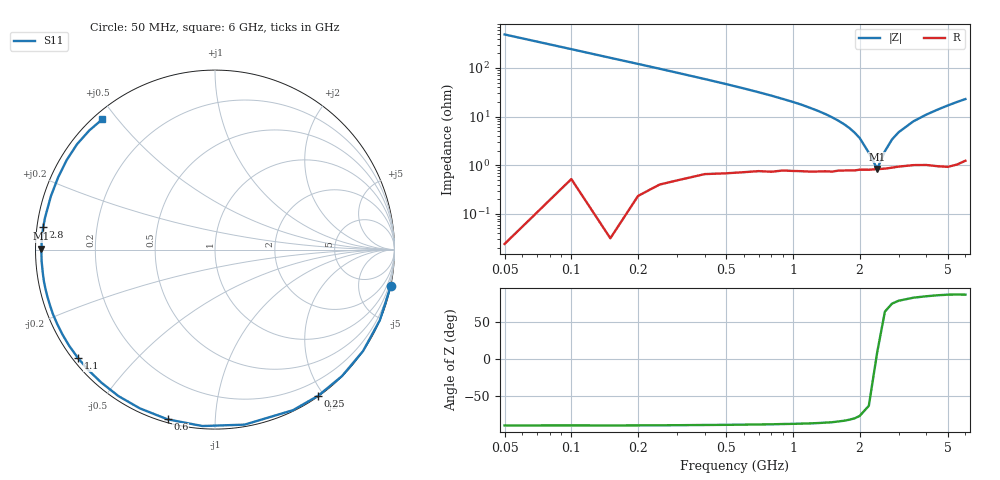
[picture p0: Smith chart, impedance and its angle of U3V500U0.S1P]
! SIEMENS Discrete & RF Semiconductors
! BBY53-02W
! Si Tuning Diode in SCD-80
! VR = 0.5 V
! S-Parameters:  September  1997
# GHz  S  MA  R  50
!  f  S11
! GHz  MAG  ANG
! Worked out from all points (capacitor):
!   34 points, 50 MHz to 6 GHz, reference 50 ohm
!   read as one part to ground: C = 6.52 pF near 50 MHz
!   lowest |Z| = 840 mohm at 2.4 GHz (marker M1)
!   series resonance near 2.385 GHz, so ESL is about 680 pH
!   S11 on the Smith chart (normalised r, x): 50 MHz: 0.00, -9.76; 250 MHz: 0.01, -1.93; 600 MHz: 0.01, -0.76; 1.1 GHz: 0.02, -0.35; 2.8 GHz: 0.02, +0.07; 6 GHz: 0.02, +0.46
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0.05  1 -11.7
0.1  0.9992 -23.2
0.15  0.9999 -34.4
0.2  0.9986 -44.9
0.25  0.9966 -54.8
0.3  0.9945 -64.1
0.4  0.9891 -80.4
0.5  0.9855 -94.1
0.6  0.9819 -105.6
0.7  0.9787 -115.3
0.8  0.9775 -123.4
0.9  0.9747 -130.5
1  0.9741 -136.4
1.1  0.9735 -141.7
1.2  0.9733 -146.6
1.3  0.9726 -150.8
1.5  0.9719 -158.1
1.6  0.9704 -161.3
1.8  0.9696 -166.9
2  0.9683 -171.9
2.4  0.9674 179.7
2.8  0.9651 172.5
3.5  0.9616 161.9
4  0.9621 155.3
4.5  0.9653 148.9
5  0.9674 142.6
5.5  0.965 136.5
6  0.9599 130.8
